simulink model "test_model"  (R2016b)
settings: Solver=VariableStepAuto  StartTime=0.0  StopTime=runtime  RelTol=1e-3
InitFcn:
  | clear mex
  | delete test_model_sfun.mexw64
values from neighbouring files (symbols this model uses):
  delta_T = 4 * [ 0,  0,  2.351e-4 ]    [modelParameters.m]
  Delta_T = cell(1,4)    [modelParameters.m]
  F_D = 1*randn(3,1)    [modelParameters.m]
  g = 9.81    [modelParameters.m]    (also in analyzeIMU_data.m = 9.8; getMomentOfInertia.m = 9.80665)
  Gamma_H = cell(1,4)    [modelParameters.m]
  have_motor_transient = 1    [modelParameters.m]
  height_controlled_o = (((Rm*If        + (((omega0_o * 2 * Rm * Kv * Kq      * Kd + 1)^2) - 1)/(4* Rm*Kv^2*Kq      * Kd))/Vb)*(Pmax - Pmin) + Pmin)    [modelParameters.m]
  i_0 = cell(1,4)    [modelParameters.m]
  If = 0.3836    [modelParameters.m]    (also in thrustDragConstantCalculations.m = [If0; If1; If2; If3]; Kd_error.m = I_0 * sign(rotor_speed_0) + I_1 * rotor_speed_0 + I_2 * roto)
  J = diag([ 0.0130 0.0140 0.0285 ])    [modelParameters.m]    (also in J_calc_bifilar.m = (16*pi^2*L./(m*g.*D.^2))\(t./n).^2)
  J_L = m_L/12*diag([y_L^2+z_L^2,x_L^2+z_L^2,x_L^2+y_L^2])    [modelParameters.m]
  J_r = cell(1,4)    [modelParameters.m]
  Jreq = 4.2012e-05    [modelParameters.m]
  Jxx = 0.0130    (= 0.013)    [modelParameters.m]
  Jyy = 0.0140    (= 0.014)    [modelParameters.m]
  Jzz = 0.0285    [modelParameters.m]
  K_d = cell(1,4)    [modelParameters.m]
  K_E = cell(1,4)    [modelParameters.m]
  K_H = cell(1,4)    [modelParameters.m]
  K_Q = cell(1,4)    [modelParameters.m]
  K_T = cell(1,4)    [modelParameters.m]
  K_V = cell(1,4)    [modelParameters.m]
  Kd = 1.4852e-07    [modelParameters.m]    (also in calcDragConstant.m = ((A'*A)^-1)*A'*b; thrustDragConstantCalculations.m = calcDragConstant(data, Pmin, Pmax, Rm, Kv, Kq, If); Kd_error.m = 1.0317e-07)
  Kh = 3.4574e-04    (= 0.00034574)    [modelParameters.m]
  Ki_mahony = 0.001    [modelParameters.m]
  Kp_mahony = 0.4    [modelParameters.m]
  Kq = 96.3422    [modelParameters.m]    (also in thrustDragConstantCalculations.m; Kd_error.m)
  Kt = 1.2007e-05    [modelParameters.m]    (also in calcThrustConstant.m = ((A'*A)^(-1))*(A'*T); thrustDragConstantCalculations.m = calcThrustConstant(data))
  Kv = 96.3422    [modelParameters.m]    (also in thrustDragConstantCalculations.m; Kd_error.m)
  m = 1.216    [modelParameters.m]
  m_L = 0    [modelParameters.m]
  omega0_o = sqrt((m*g)/(4*Kt))    [modelParameters.m]
  omega1_o = sqrt((m*g)/(4*Kt))    [modelParameters.m]
  omega2_o = sqrt((m*g)/(4*Kt))    [modelParameters.m]
  omega3_o = sqrt((m*g)/(4*Kt))    [modelParameters.m]
  omega_0 = cell(1,4)    [modelParameters.m]
  p0 = 0    [modelParameters.m]
  p_0 = cell(1,4)    [modelParameters.m]
  p_max = cell(1,4)    [modelParameters.m]
  phi0 = 0    [modelParameters.m]
  pitch_o = 0    [modelParameters.m]
  pitchrate_o = 0    [modelParameters.m]
  Pmax = 1    [modelParameters.m]    (also in thrustDragConstantCalculations.m = 200000; Kd_error.m = 200000)
  Pmin = 0    [modelParameters.m]    (also in thrustDragConstantCalculations.m = 100000; Kd_error.m = 100000)
  psi0 = 0    [modelParameters.m]
  q0 = 0    [modelParameters.m]
  Q_D = 0.05*randn(3,1)    [modelParameters.m]
  r0 = 0    [modelParameters.m]
  R_m = cell(1,4)    [modelParameters.m]
  r_oc = [ 0 ; 0 ; 0 ]    [modelParameters.m]
  r_oL = [0; 0; 0]    [modelParameters.m]
  rhx = 0.16    [modelParameters.m]
  rhy = 0.16    [modelParameters.m]
  rhz = 0.03    [modelParameters.m]
  Rm = 0.235    [modelParameters.m]    (also in thrustDragConstantCalculations.m = 0.2308; Kd_error.m = 0.2308)
  roll_o = 0    [modelParameters.m]
  rollrate_o = 0    [modelParameters.m]
  Tc = 0.04    [modelParameters.m]
  theta0 = 0    [modelParameters.m]
  Tq = 0.005    [modelParameters.m]
  u0 = 0    [modelParameters.m]
  v0 = 0    [modelParameters.m]
  Vb = 12.3    [modelParameters.m]    (also in calcDragConstant.m = [data.(6); data.(6); data.(6); data.(6)]; Kd_error.m = data.(6))
  w0 = 0    [modelParameters.m]
  x0 = 0    [modelParameters.m]
  x_controlled_o = 0    [modelParameters.m]
  x_o = 0    [modelParameters.m]
  x_vel_o = 0    [modelParameters.m]
  y0 = 0    [modelParameters.m]
  y_controlled_o = 0    [modelParameters.m]
  y_o = 0    [modelParameters.m]
  y_vel_o = 0    [modelParameters.m]
  yaw_controlled_o = 0    [modelParameters.m]
  yaw_o = 0    [modelParameters.m]
  yawrate_o = 0    [modelParameters.m]
  z0 = 0    [modelParameters.m]
  z_o = 0    [modelParameters.m]
  z_vel_o = 0    [modelParameters.m]
undefined symbols (not defined in the file or in its folder): Gamma_Omega, Gamma_T, Ki, Kp, r_h, slope, start, Ts, X0
libraries: simulink x32, Derivative x26, dsparch4 x6, vrlib x4
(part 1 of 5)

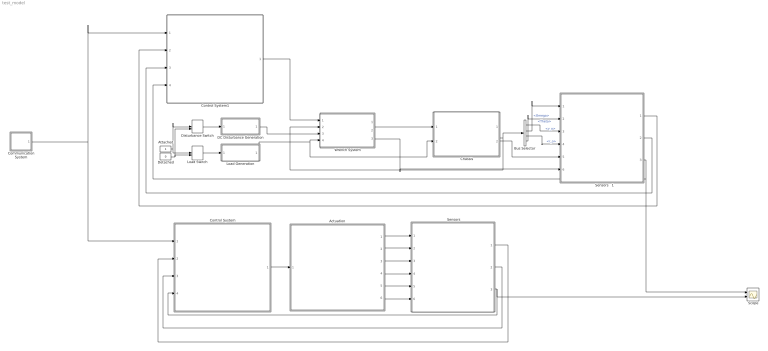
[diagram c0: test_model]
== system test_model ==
  "     Sensors   " : Subsystem
  "     Sensors   1" : Subsystem
  Actuation : Subsystem
  Attached : Constant
  Bus Selector : BusSelector  OutputSignals=v_o,Omega,r_o,Theta
  Chassis : Subsystem
  Communication System : Subsystem
  Control System : Subsystem
  Control System1 : Subsystem
  DC Disturbance Generation : Subsystem
  Detached : Constant  Value=0
  Disturbance Switch : ManualSwitch  CurrentSetting=0
  Load Generation : Subsystem
  Load Switch : ManualSwitch  CurrentSetting=0
  Scope : Scope  NumInputPorts=2
  Wrench System : Subsystem
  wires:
  Communication System/1(setpoints) -> Control System1/1(setpoints), Control System/1(setpoints)
  Wrench System/1(W) -> Chassis/1(W)
  Load Generation/1(Load) -> Chassis/2(Load), Wrench System/4(Load)
  DC Disturbance Generation/1(Disturbance) -> Wrench System/3(W_D)
  Attached/1 -> Load Switch/1, Disturbance Switch/1
  Detached/1 -> Load Switch/2, Disturbance Switch/2
  Load Switch/1 -> Load Generation/1(On/Off)
  Disturbance Switch/1 -> DC Disturbance Generation/1(On/Off)
  Chassis/1(Lambda) -> Wrench System/2(Lambda), Bus Selector/1
  Control System1/1(P) -> Wrench System/1(P)
  Control System/1(P) -> Actuation/1(P)
  Actuation/6(B_g) -> "     Sensors   "/6(B_g)
  Actuation/5(B_vo_dot) -> "     Sensors   "/5(B_vo_dot)
  Actuation/4(E_ro) -> "     Sensors   "/4(E_ro)
  Actuation/3(B_vo) -> "     Sensors   "/3(B_vo)
  Actuation/1(B_omega) -> "     Sensors   "/1(B_Omega)
  "     Sensors   "/3(current_position) -> Control System/4(current_position), Scope/2
  "     Sensors   "/2(euler_rates) -> Control System/3(euler_rates)
  "     Sensors   "/1(euler_angles_filtered) -> Control System/2(euler_angles_filtered)
  Bus Selector/1 -> "     Sensors   1"/3(B_vo)  "<v_o>"
  Bus Selector/2 -> "     Sensors   1"/1(B_Omega)  "<Omega>"
  Bus Selector/3 -> "     Sensors   1"/4(E_ro)  "<r_o>"
  Bus Selector/4 -> "     Sensors   1"/2(euler_angles)  "<Theta>"
  Chassis/2(B_vo_dot) -> "     Sensors   1"/5(B_vo_dot)
  Wrench System/3(Bg) -> "     Sensors   1"/6(B_g)
  "     Sensors   1"/3(current_position) -> Control System1/4(current_position), Scope/1
  "     Sensors   1"/2(euler_rates) -> Control System1/3(euler_rates)
  "     Sensors   1"/1(euler_angles_filtered) -> Control System1/2(euler_angles_filtered)
  Actuation/2(euler_angles) -> "     Sensors   "/2(euler_angles)

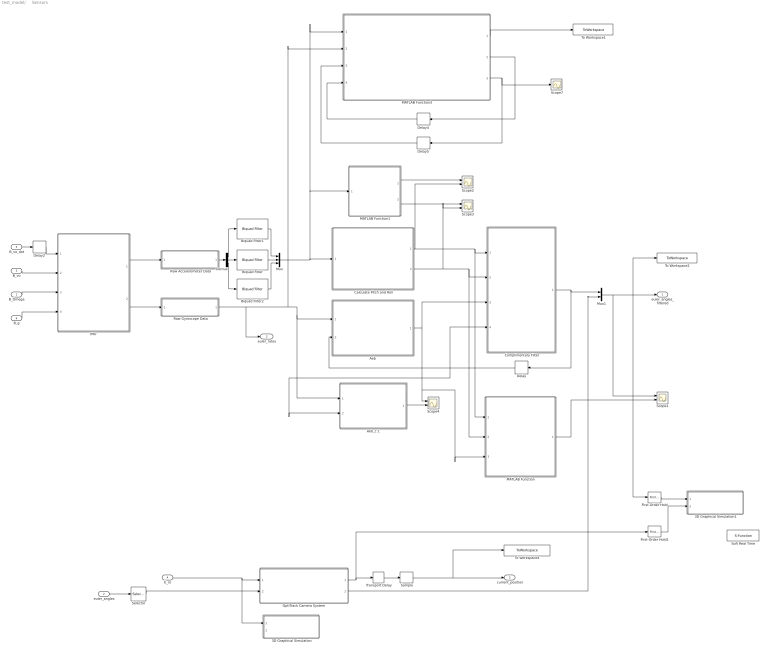
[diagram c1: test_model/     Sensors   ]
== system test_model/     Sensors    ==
  B_Omega : Inport
  euler_angles : Inport  Port=2
  B_vo : Inport  Port=3
  E_ro : Inport  Port=4
  B_vo_dot : Inport  Port=5
  B_g : Inport  Port=6
  3D Graphical Simulation : Subsystem  Commented=on
  3D Graphical Simulation1 : Subsystem  Commented=on
  "Aeb " : MATLAB Function  TreatAsAtomicUnit=on
  Aeb_c 1 : MATLAB Function  TreatAsAtomicUnit=on
  Biquad Filter : dsparch4/Biquad Filter  IIRFiltStruct=Direct form II  CoeffSource=Specify via dialog  BiQuadCoeffs=SOS_Matrix  a0Flag=Warning  IC=0  ICnum=0  ICden=0  InputProcessing=Columns as channels (frame based)  denAccumFracLength=30  denProdOutputFracLength=30  secondMemoryFracLength=15  roundingMode=Floor  overflowMode=off  ScaleValues=1  optimizeScaleValues=on  ScaleValueMode=Specify via input port (g)  scaleValueFracLength=14  FilterSource=Specify via dialog  FilterObject=BQF
  Biquad Filter1 : dsparch4/Biquad Filter  IIRFiltStruct=Direct form II  CoeffSource=Specify via dialog  BiQuadCoeffs=SOS_Matrix  a0Flag=Warning  IC=0  ICnum=0  ICden=0  InputProcessing=Columns as channels (frame based)  denAccumFracLength=30  denProdOutputFracLength=30  secondMemoryFracLength=15  roundingMode=Floor  overflowMode=off  ScaleValues=1  optimizeScaleValues=on  ScaleValueMode=Specify via input port (g)  scaleValueFracLength=14  FilterSource=Specify via dialog  FilterObject=BQF
  Biquad Filter2 : dsparch4/Biquad Filter  IIRFiltStruct=Direct form II  CoeffSource=Specify via dialog  BiQuadCoeffs=SOS_Matrix  a0Flag=Warning  IC=0  ICnum=0  ICden=0  InputProcessing=Columns as channels (frame based)  denAccumFracLength=30  denProdOutputFracLength=30  secondMemoryFracLength=15  roundingMode=Floor  overflowMode=off  ScaleValues=1  optimizeScaleValues=on  ScaleValueMode=Specify via input port (g)  scaleValueFracLength=14  FilterSource=Specify via dialog  FilterObject=BQF
  Calculate Pitch and Roll : MATLAB Function  TreatAsAtomicUnit=on
  Complimentary Filter : MATLAB Function  TreatAsAtomicUnit=on
  Delay : Delay  DelayLength=1  InitialCondition=0
  Delay2 : Delay  DelayLength=1  InitialCondition=0  SampleTime=Tq
  Delay4 : Delay  DelayLength=1  InitialCondition=0  SampleTime=Tq
  Delay5 : Delay  DelayLength=1  InitialCondition=[1, 0, 0, 0]  SampleTime=Tq
  Demux : Demux  Outputs=3
  First-Order Hold : simulink/Discrete/First-Order Hold  DisableCoverage=on  Ts=5e-3
  First-Order Hold1 : simulink/Discrete/First-Order Hold  DisableCoverage=on  Ts=5e-3
  "IMU " : Subsystem
  MATLAB Function : MATLAB Function  TreatAsAtomicUnit=on
  MATLAB Function1 : MATLAB Function  TreatAsAtomicUnit=on
  MATLAB Function3 : MATLAB Function  TreatAsAtomicUnit=on
  Mux : Mux  Inputs=3
  Mux1 : Mux  Inputs=2
  "OptiTrack Camera System " : Subsystem
  Raw Accelerometer Data : Subsystem  Variant=on
  Raw Gyroscope Data : Subsystem  Variant=on
  Sample : ZeroOrderHold  SampleTime=Tc
  Scope{1..4} (4 alike) : Scope  NumInputPorts=2
  Scope7 : Scope
  Selector : Selector  InputPortWidth=3  IndexOptions=Index vector (dialog)  Indices=[3]  OutputSizes=1
  Soft Real Time : S-Function  Commented=on  FunctionName=sfun_time  Parameters=x  SFunctionDeploymentMode=off  EnableBusSupport=off
  To Workspace1 : ToWorkspace  VariableName=mahony_reading  SaveFormat=Structure With Time  SampleTime=Tq
  To Workspace2 : ToWorkspace  VariableName=angle_IMU_reading  SaveFormat=Structure With Time  SampleTime=Tq
  To Workspace4 : ToWorkspace  VariableName=position_model  SaveFormat=Structure With Time  SampleTime=Tc
  Transport Delay : TransportDelay  DelayTime=6e-3
  euler_angles_filtered : Outport
  euler_rates : Outport  Port=2
  current_position : Outport  Port=3
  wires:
  "IMU "/1(accelerometer) -> Raw Accelerometer Data/1(raw_accel_model)
  "IMU "/2(gyroscope) -> Raw Gyroscope Data/1(raw_gyro_model)
  B_vo/1 -> "IMU "/2(B_vo)
  B_Omega/1 -> "IMU "/3(B_Omega)
  B_g/1 -> "IMU "/4(B_g)
  Calculate Pitch and Roll/2(accel_roll) -> Scope3/2, MATLAB Function/2(accel_roll), Complimentary Filter/2(accel_roll)
  Calculate Pitch and Roll/1(accel_pitch) -> MATLAB Function/1(accel_pitch), Complimentary Filter/1(accel_pitch), Scope2/2
  First-Order Hold/1 -> 3D Graphical Simulation1/1("Euler Angles ")
  E_ro/1 -> 3D Graphical Simulation/1(Displacement), "OptiTrack Camera System "/1(E_ro)
  First-Order Hold1/1 -> 3D Graphical Simulation1/2(Displacement)
  B_vo_dot/1 -> Delay2/1
  Delay2/1 -> "IMU "/1(B_vo_dot)
  "OptiTrack Camera System "/1(E_ro_camera) -> Transport Delay/1, First-Order Hold1/1
  Transport Delay/1 -> Sample/1
  Sample/1 -> To Workspace4/1, current_position/1
  Raw Gyroscope Data/1(raw_gyro) -> Aeb_c 1/1(gyro_reading), "Aeb "/1(gyro_reading), MATLAB Function3/2(gyroReadings), euler_rates/1
  Delay/1 -> Complimentary Filter/4(prev_euler_angles), Aeb_c 1/2(euler_angles_filtered), "Aeb "/2(euler_angles_filtered)
  Aeb_c 1/1(euler_rates_IMU) -> Scope4/2
  MATLAB Function1/1(accel_pitch) -> Scope2/1
  MATLAB Function1/2(accel_roll) -> Scope3/1
  "OptiTrack Camera System "/2(yaw_camera) -> Mux1/2
  MATLAB Function3/1(eulerAngles) -> To Workspace1/1
  MATLAB Function3/2(integralFeedback) -> Delay4/1
  Delay4/1 -> MATLAB Function3/4(integralFeedback_prev)
  MATLAB Function3/3(quaternions) -> Scope7/1, Delay5/1
  Delay5/1 -> MATLAB Function3/3(quaternions_prev)
  "Aeb "/1(euler_rates_IMU) -> MATLAB Function/3(euler_rates_gyro), Scope4/1, Complimentary Filter/3(euler_rates_gyro)
  Raw Accelerometer Data/1(raw_accel) -> Demux/1
  Demux/2 -> Biquad Filter/1
  Demux/1 -> Biquad Filter1/1
  Demux/3 -> Biquad Filter2/1
  Biquad Filter/1 -> Mux/2
  Biquad Filter1/1 -> Mux/1
  Biquad Filter2/1 -> Mux/3
  Mux/1 -> Calculate Pitch and Roll/1(accel_reading), MATLAB Function1/1(accel_reading), MATLAB Function3/1(accelReadings)
  Complimentary Filter/1(euler_angles_IMU) -> Mux1/1, Delay/1
  euler_angles/1 -> Selector/1
  Selector/1 -> "OptiTrack Camera System "/2(yaw)
  MATLAB Function/1(euler_angles_IMU) -> Scope1/2
  Mux1/1 -> Scope1/1, To Workspace2/1, First-Order Hold/1, euler_angles_filtered/1

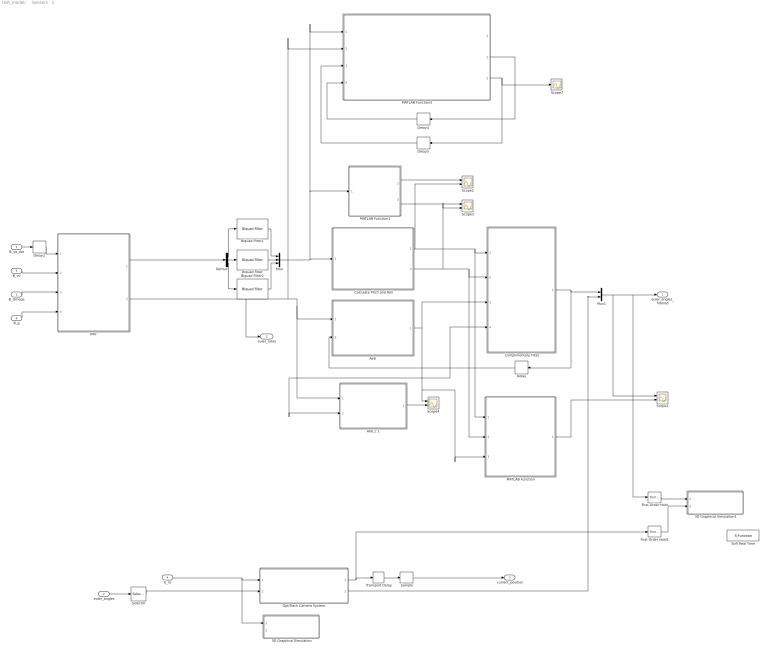
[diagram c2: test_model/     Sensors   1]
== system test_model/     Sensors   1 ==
  B_Omega : Inport
  euler_angles : Inport  Port=2
  B_vo : Inport  Port=3
  E_ro : Inport  Port=4
  B_vo_dot : Inport  Port=5
  B_g : Inport  Port=6
  3D Graphical Simulation : Subsystem  Commented=on
  3D Graphical Simulation1 : Subsystem  Commented=on
  "Aeb " : MATLAB Function  TreatAsAtomicUnit=on
  Aeb_c 1 : MATLAB Function  TreatAsAtomicUnit=on
  Biquad Filter : dsparch4/Biquad Filter  IIRFiltStruct=Direct form II  CoeffSource=Specify via dialog  BiQuadCoeffs=SOS_Matrix  a0Flag=Warning  IC=0  ICnum=0  ICden=0  InputProcessing=Columns as channels (frame based)  denAccumFracLength=30  denProdOutputFracLength=30  secondMemoryFracLength=15  roundingMode=Floor  overflowMode=off  ScaleValues=1  optimizeScaleValues=on  ScaleValueMode=Specify via input port (g)  scaleValueFracLength=14  FilterSource=Specify via dialog  FilterObject=BQF
  Biquad Filter1 : dsparch4/Biquad Filter  IIRFiltStruct=Direct form II  CoeffSource=Specify via dialog  BiQuadCoeffs=SOS_Matrix  a0Flag=Warning  IC=0  ICnum=0  ICden=0  InputProcessing=Columns as channels (frame based)  denAccumFracLength=30  denProdOutputFracLength=30  secondMemoryFracLength=15  roundingMode=Floor  overflowMode=off  ScaleValues=1  optimizeScaleValues=on  ScaleValueMode=Specify via input port (g)  scaleValueFracLength=14  FilterSource=Specify via dialog  FilterObject=BQF
  Biquad Filter2 : dsparch4/Biquad Filter  IIRFiltStruct=Direct form II  CoeffSource=Specify via dialog  BiQuadCoeffs=SOS_Matrix  a0Flag=Warning  IC=0  ICnum=0  ICden=0  InputProcessing=Columns as channels (frame based)  denAccumFracLength=30  denProdOutputFracLength=30  secondMemoryFracLength=15  roundingMode=Floor  overflowMode=off  ScaleValues=1  optimizeScaleValues=on  ScaleValueMode=Specify via input port (g)  scaleValueFracLength=14  FilterSource=Specify via dialog  FilterObject=BQF
  Calculate Pitch and Roll : MATLAB Function  TreatAsAtomicUnit=on
  Complimentary Filter : MATLAB Function  TreatAsAtomicUnit=on
  Delay : Delay  DelayLength=1  InitialCondition=0
  Delay2 : Delay  DelayLength=1  InitialCondition=0  SampleTime=Tq
  Delay4 : Delay  DelayLength=1  InitialCondition=0  SampleTime=Tq
  Delay5 : Delay  DelayLength=1  InitialCondition=[1, 0, 0, 0]  SampleTime=Tq
  Demux : Demux  Outputs=3
  First-Order Hold : simulink/Discrete/First-Order Hold  DisableCoverage=on  Ts=5e-3
  First-Order Hold1 : simulink/Discrete/First-Order Hold  DisableCoverage=on  Ts=5e-3
  "IMU " : Subsystem
  MATLAB Function : MATLAB Function  TreatAsAtomicUnit=on
  MATLAB Function1 : MATLAB Function  TreatAsAtomicUnit=on
  MATLAB Function3 : MATLAB Function  TreatAsAtomicUnit=on
  Mux : Mux  Inputs=3
  Mux1 : Mux  Inputs=2
  "OptiTrack Camera System " : Subsystem
  Sample : ZeroOrderHold  SampleTime=Tc
  Scope{1..4} (4 alike) : Scope  NumInputPorts=2
  Scope7 : Scope
  Selector : Selector  InputPortWidth=3  IndexOptions=Index vector (dialog)  Indices=[3]  OutputSizes=1
  Soft Real Time : S-Function  Commented=on  FunctionName=sfun_time  Parameters=x  SFunctionDeploymentMode=off  EnableBusSupport=off
  Transport Delay : TransportDelay  DelayTime=6e-3
  euler_angles_filtered : Outport
  euler_rates : Outport  Port=2
  current_position : Outport  Port=3
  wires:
  B_vo/1 -> "IMU "/2(B_vo)
  B_Omega/1 -> "IMU "/3(B_Omega)
  B_g/1 -> "IMU "/4(B_g)
  Calculate Pitch and Roll/2(accel_roll) -> Scope3/2, MATLAB Function/2(accel_roll), Complimentary Filter/2(accel_roll)
  Calculate Pitch and Roll/1(accel_pitch) -> MATLAB Function/1(accel_pitch), Complimentary Filter/1(accel_pitch), Scope2/2
  First-Order Hold/1 -> 3D Graphical Simulation1/1("Euler Angles ")
  E_ro/1 -> 3D Graphical Simulation/1(Displacement), "OptiTrack Camera System "/1(E_ro)
  First-Order Hold1/1 -> 3D Graphical Simulation1/2(Displacement)
  B_vo_dot/1 -> Delay2/1
  Delay2/1 -> "IMU "/1(B_vo_dot)
  "OptiTrack Camera System "/1(E_ro_camera) -> Transport Delay/1, First-Order Hold1/1
  Transport Delay/1 -> Sample/1
  Sample/1 -> current_position/1
  "IMU "/2(gyroscope) -> Aeb_c 1/1(gyro_reading), "Aeb "/1(gyro_reading), MATLAB Function3/2(gyroReadings), euler_rates/1
  Delay/1 -> Complimentary Filter/4(prev_euler_angles), Aeb_c 1/2(euler_angles_filtered), "Aeb "/2(euler_angles_filtered)
  Aeb_c 1/1(euler_rates_IMU) -> Scope4/2
  MATLAB Function1/1(accel_pitch) -> Scope2/1
  MATLAB Function1/2(accel_roll) -> Scope3/1
  "OptiTrack Camera System "/2(yaw_camera) -> Mux1/2
  MATLAB Function3/2(integralFeedback) -> Delay4/1
  Delay4/1 -> MATLAB Function3/4(integralFeedback_prev)
  MATLAB Function3/3(quaternions) -> Scope7/1, Delay5/1
  Delay5/1 -> MATLAB Function3/3(quaternions_prev)
  "Aeb "/1(euler_rates_IMU) -> MATLAB Function/3(euler_rates_gyro), Scope4/1, Complimentary Filter/3(euler_rates_gyro)
  "IMU "/1(accelerometer) -> Demux/1
  Demux/2 -> Biquad Filter/1
  Demux/1 -> Biquad Filter1/1
  Demux/3 -> Biquad Filter2/1
  Biquad Filter/1 -> Mux/2
  Biquad Filter1/1 -> Mux/1
  Biquad Filter2/1 -> Mux/3
  Mux/1 -> Calculate Pitch and Roll/1(accel_reading), MATLAB Function1/1(accel_reading), MATLAB Function3/1(accelReadings)
  Complimentary Filter/1(euler_angles_IMU) -> Mux1/1, Delay/1
  euler_angles/1 -> Selector/1
  Selector/1 -> "OptiTrack Camera System "/2(yaw)
  MATLAB Function/1(euler_angles_IMU) -> Scope1/2
  Mux1/1 -> Scope1/1, First-Order Hold/1, euler_angles_filtered/1

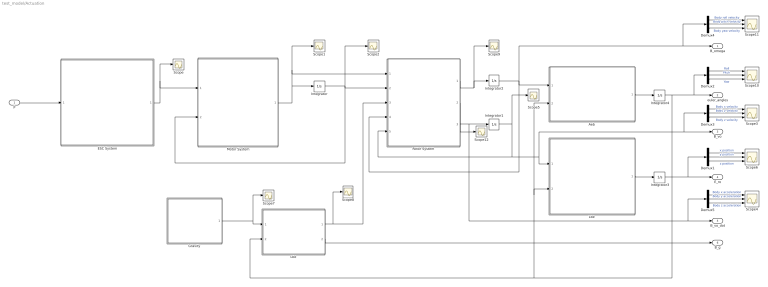
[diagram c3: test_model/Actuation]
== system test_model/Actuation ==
  P : Inport
  "Aeb " : MATLAB Function  TreatAsAtomicUnit=on
  Demux{1..5} (5 alike) : Demux  Outputs=3
  ESC System : MATLAB Function  TreatAsAtomicUnit=on
  "Gravity " : MATLAB Function  TreatAsAtomicUnit=on
  Integrator : Integrator  InitialCondition=[omega0_o, omega1_o, omega2_o, omega3_o]
  Integrator1 : Integrator  InitialCondition=[x_vel_o; y_vel_o; z_vel_o]
  Integrator2 : Integrator  InitialCondition=[rollrate_o; pitchrate_o; yawrate_o]
  Integrator3 : Integrator  InitialCondition=[x_o; y_o; z_o]
  Integrator4 : Integrator  InitialCondition=[roll_o; pitch_o; yaw_o]  ContinuousStateAttributes=['phi' 'theta' 'psi']
  "Lbe " : MATLAB Function  TreatAsAtomicUnit=on
  "Lbe " : MATLAB Function  TreatAsAtomicUnit=on
  Motor System : MATLAB Function  TreatAsAtomicUnit=on
  "Rotor System " : MATLAB Function  TreatAsAtomicUnit=on
  Scope{,1..2,5,7..9,12} (8 alike) : Scope
  Scope{3..4,6,10..11} (5 alike) : Scope  NumInputPorts=3
  B_omega : Outport
  euler_angles : Outport  Port=2
  B_vo : Outport  Port=3
  E_ro : Outport  Port=4
  B_vo_dot : Outport  Port=5
  B_g : Outport  Port=6
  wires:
  ESC System/1(Vb_eff) -> Scope/1, Motor System/1(Vb_eff)
  "Rotor System "/1(B_omega_dot) -> Scope9/1, Integrator2/1
  Integrator2/1 -> "Rotor System "/4(B_omega), B_omega/1, Demux4/1, "Aeb "/1(B_omega)
  "Aeb "/1(euler_rates) -> Integrator4/1
  "Lbe "/1(E_ro) -> Integrator3/1
  Integrator3/1 -> Demux1/1, E_ro/1
  "Lbe "/1(B_Fg) -> Scope8/1, "Rotor System "/3(B_Fg)
  "Lbe "/2(B_g) -> B_g/1
  Demux1/2 -> Scope6/2  "y position"
  Demux1/1 -> Scope6/1  "x position"
  Demux1/3 -> Scope6/3  "z position"
  Demux2/2 -> Scope10/2  "Pitch"
  Demux2/1 -> Scope10/1  "Roll"
  Demux2/3 -> Scope10/3  "Yaw"
  Demux4/2 -> Scope11/2  "Body pitch velocity"
  Demux4/1 -> Scope11/1  "Body roll velocity"
  Demux4/3 -> Scope11/3  "Body yaw velocity"
  Demux3/2 -> Scope3/2  "Body y velocity"
  Demux3/1 -> Scope3/1  "Body x velocity"
  Demux3/3 -> Scope3/3  "Body z velocity"
  Demux5/2 -> Scope4/2  "Body y acceleration"
  Demux5/1 -> Scope4/1  "Body x acceleration"
  Demux5/3 -> Scope4/3  "Body z acceleration"
  Integrator1/1 -> Scope5/1, "Rotor System "/5(B_vo), "Lbe "/1(B_vo), Demux3/1, B_vo/1
  "Rotor System "/2(B_vo_dot) -> Demux5/1, B_vo_dot/1, Integrator1/1
  Integrator4/1 -> euler_angles/1, Demux2/1, "Lbe "/2(euler_angles), "Aeb "/2(euler_angles), "Lbe "/2(euler_angles)
  P/1 -> ESC System/1(P)
  "Gravity "/1(E_Fg) -> Scope7/1, "Lbe "/1(E_Fg)
  Integrator/1 -> Motor System/2(w), "Rotor System "/2(w), Scope2/1
  Motor System/1(w_dot) -> Integrator/1, Scope1/1, "Rotor System "/1(w_dot)
  "Rotor System "/3(B_F) -> Scope12/1

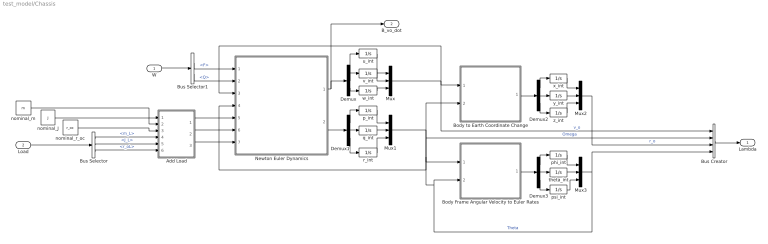
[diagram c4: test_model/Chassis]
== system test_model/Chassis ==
  W : Inport
  Load : Inport  Port=2
  Add Load : Subsystem
  Body Frame Angular Velocity to Euler Rates : MATLAB Function  TreatAsAtomicUnit=on
  Body to Earth Coordinate Change : MATLAB Function  TreatAsAtomicUnit=on
  Bus Creator : BusCreator  Inputs=4
  Bus Selector : BusSelector  OutputSignals=m_L,J_L,r_oL
  Bus Selector1 : BusSelector  OutputSignals=F,Q
  Demux{,1..3} (4 alike) : Demux  Outputs=3
  Mux{,1..3} (4 alike) : Mux  Inputs=3
  Newton Euler Dynamics : Subsystem
  nominal_J : Constant  Value=J
  nominal_m : Constant  Value=m
  nominal_r_oc : Constant  Value=r_oc
  p_int : Integrator  InitialCondition=p0  ContinuousStateAttributes='p'
  phi_int : Integrator  InitialCondition=phi0  ContinuousStateAttributes='phi'
  psi_int : Integrator  InitialCondition=psi0  ContinuousStateAttributes='psi'
  q_int : Integrator  InitialCondition=q0  ContinuousStateAttributes='q'
  r_int : Integrator  InitialCondition=r0  ContinuousStateAttributes='r'
  theta_int : Integrator  InitialCondition=theta0  ContinuousStateAttributes='theta'
  u_int : Integrator  InitialCondition=u0  ContinuousStateAttributes='u'
  v_int : Integrator  InitialCondition=v0  ContinuousStateAttributes='v'
  w_int : Integrator  InitialCondition=w0  ContinuousStateAttributes='w'
  x_int : Integrator  InitialCondition=x0  ContinuousStateAttributes='x'
  y_int : Integrator  InitialCondition=y0  ContinuousStateAttributes='y'
  z_int : Integrator  InitialCondition=z0  ContinuousStateAttributes='z'
  Lambda : Outport
  B_vo_dot : Outport  Port=2
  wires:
  nominal_J/1 -> Add Load/2(J_0)
  Bus Selector/3 -> Add Load/6(r_ol)  "<r_oL>"
  Bus Selector/2 -> Add Load/5(J_l)  "<J_L>"
  Bus Selector/1 -> Add Load/4(m_l)  "<m_L>"
  Add Load/3(r_oc) -> Newton Euler Dynamics/7(r_oc)
  Add Load/2(J) -> Newton Euler Dynamics/6(J)
  Add Load/1(m) -> Newton Euler Dynamics/5(m)
  W/1 -> Bus Selector1/1
  Bus Selector1/2 -> Newton Euler Dynamics/2(Q)  "<Q>"
  Bus Selector1/1 -> Newton Euler Dynamics/1(F)  "<F>"
  Body Frame Angular Velocity to Euler Rates/1(dot_Theta) -> Demux3/1
  Demux3/3 -> psi_int/1
  Demux3/2 -> theta_int/1
  Demux3/1 -> phi_int/1
  psi_int/1 -> Mux3/3
  theta_int/1 -> Mux3/2
  phi_int/1 -> Mux3/1
  Body to Earth Coordinate Change/1(x_E) -> Demux2/1
  Demux2/3 -> z_int/1
  Demux2/2 -> y_int/1
  Demux2/1 -> x_int/1
  z_int/1 -> Mux2/3
  y_int/1 -> Mux2/2
  x_int/1 -> Mux2/1
  Newton Euler Dynamics/2(dOmega) -> Demux1/1
  Demux1/3 -> r_int/1
  Demux1/2 -> q_int/1
  Demux1/1 -> p_int/1
  r_int/1 -> Mux1/3
  q_int/1 -> Mux1/2
  p_int/1 -> Mux1/1
  Newton Euler Dynamics/1(dv) -> B_vo_dot/1, Demux/1
  Demux/3 -> w_int/1
  Demux/2 -> v_int/1
  Demux/1 -> u_int/1
  w_int/1 -> Mux/3
  v_int/1 -> Mux/2
  u_int/1 -> Mux/1
  Bus Creator/1 -> Lambda/1
  Mux3/1 -> Body to Earth Coordinate Change/2(Theta), Body Frame Angular Velocity to Euler Rates/2(Theta), Bus Creator/4  "Theta"
  Mux2/1 -> Bus Creator/3  "r_o"
  Mux1/1 -> Body Frame Angular Velocity to Euler Rates/1(Omega_B), Newton Euler Dynamics/4(Omega), Bus Creator/2  "Omega"
  Mux/1 -> Bus Creator/1, Body to Earth Coordinate Change/1(x_B), Newton Euler Dynamics/3(v)  "v_o"
  nominal_m/1 -> Add Load/1(m_0)
  nominal_r_oc/1 -> Add Load/3(r_oc_0)
  Load/1 -> Bus Selector/1

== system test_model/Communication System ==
  From Workspace : FromWorkspace  VariableName=x_setpoint_model  SampleTime=Tq  Interpolate=off  OutputAfterFinalValue=Holding final value
  From Workspace1 : FromWorkspace  VariableName=z_setpoint_model  SampleTime=Tq  Interpolate=off  OutputAfterFinalValue=Holding final value
  From Workspace2 : FromWorkspace  VariableName=y_setpoint_model  SampleTime=Tq  Interpolate=off  OutputAfterFinalValue=Holding final value
  Mux : Mux
  Step : Step  Before=[0; 0; 0; 0]  After=[0; 0; 1; 0]  SampleTime=Tq
  Step1 : Step  After=0  SampleTime=0
  setpoints : Outport
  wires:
  From Workspace/1 -> Mux/1
  Mux/1 -> setpoints/1
  From Workspace2/1 -> Mux/2
  From Workspace1/1 -> Mux/3
  Step1/1 -> Mux/4

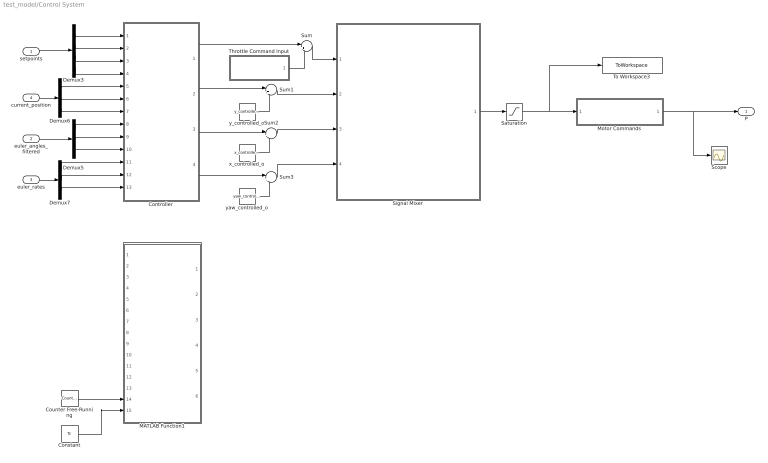
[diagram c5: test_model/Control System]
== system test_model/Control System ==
  setpoints : Inport
  euler_angles_filtered : Inport  Port=2
  euler_rates : Inport  Port=3
  current_position : Inport  Port=4
  Constant : Constant  Value=Tc  SampleTime=Tc
  Controller : Subsystem
  Counter Free-Running : simulink/Sources/Counter Free-Running  NumBits=32  tsamp=Tc
  Demux3 : Demux
  Demux5 : Demux  Outputs=3
  Demux6 : Demux  Outputs=3
  Demux7 : Demux  Outputs=3
  MATLAB Function1 : MATLAB Function  Commented=on  TreatAsAtomicUnit=on  SystemSampleTime=Tq
  Motor Commands : Subsystem  Commented=through  Variant=on
  Saturation : Saturate  UpperLimit=Pmax*ones(4,1)  LowerLimit=Pmin*ones(4,1)
  Scope : Scope
  Signal Mixer : MATLAB Function  TreatAsAtomicUnit=on
  Sum{,1..3} (4 alike) : Sum  Inputs=|++
  Throttle Command Input : Subsystem  Variant=on
  To Workspace3 : ToWorkspace  VariableName=motorCommands  SaveFormat=Structure With Time  SampleTime=Tq
  x_controlled_o : Constant  Value=x_controlled_o
  y_controlled_o : Constant  Value=y_controlled_o
  yaw_controlled_o : Constant  Value=yaw_controlled_o
  P : Outport
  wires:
  y_controlled_o/1 -> Sum1/2
  x_controlled_o/1 -> Sum2/2
  yaw_controlled_o/1 -> Sum3/2
  Signal Mixer/1(P) -> Saturation/1
  Counter Free-Running/1 -> MATLAB Function1/14(vrpn_id)
  Constant/1 -> MATLAB Function1/15(Tc)
  Sum1/1 -> Signal Mixer/2(y_controlled)
  Sum2/1 -> Signal Mixer/3(x_controlled)
  Sum3/1 -> Signal Mixer/4(yaw_controlled)
  Motor Commands/1(z_command) -> P/1, Scope/1
  Saturation/1 -> To Workspace3/1, Motor Commands/1(z_command_model)
  setpoints/1 -> Demux3/1
  current_position/1 -> Demux6/1
  euler_angles_filtered/1 -> Demux5/1
  euler_rates/1 -> Demux7/1
  Demux3/1 -> Controller/1(x_setpoint)
  Demux3/2 -> Controller/2(y_setpoint)
  Demux3/3 -> Controller/3(z_setpoint)
  Demux3/4 -> Controller/4(yaw_setpoint)
  Demux6/1 -> Controller/5(x_position)
  Demux6/2 -> Controller/6(y_position)
  Demux6/3 -> Controller/7(z_position)
  Demux5/1 -> Controller/8(roll)
  Demux5/2 -> Controller/9(pitch)
  Demux5/3 -> Controller/10(yaw)
  Demux7/1 -> Controller/11(roll_rate)
  Demux7/2 -> Controller/12(pitch_rate)
  Demux7/3 -> Controller/13(yaw_rate)
  Controller/1(height_controlled) -> Sum/1
  Controller/2(y_controlled) -> Sum1/1
  Controller/3(x_controlled) -> Sum2/1
  Controller/4(yaw_controlled) -> Sum3/1
  Throttle Command Input/1(z_command) -> Sum/2
  Sum/1 -> Signal Mixer/1(height_controlled)

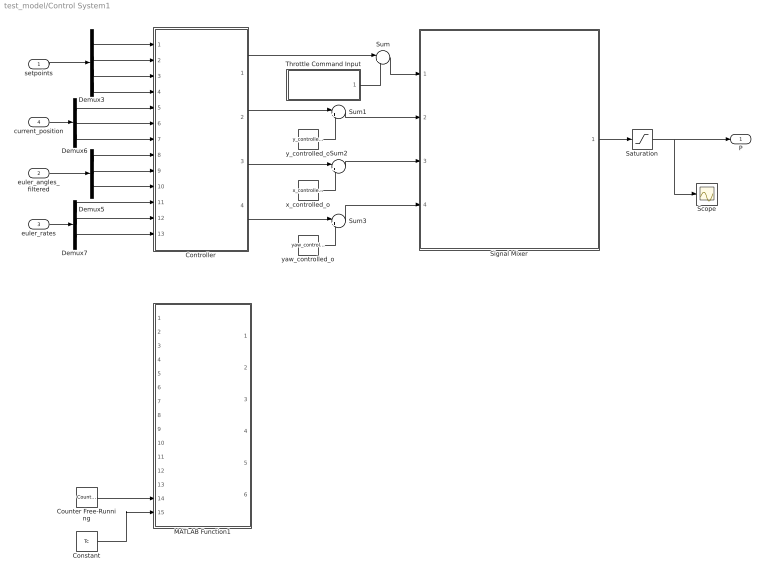
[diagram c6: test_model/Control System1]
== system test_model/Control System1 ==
  setpoints : Inport
  euler_angles_filtered : Inport  Port=2
  euler_rates : Inport  Port=3
  current_position : Inport  Port=4
  Constant : Constant  Value=Tc  SampleTime=Tc
  Controller : Subsystem
  Counter Free-Running : simulink/Sources/Counter Free-Running  NumBits=32  tsamp=Tc
  Demux3 : Demux
  Demux5 : Demux  Outputs=3
  Demux6 : Demux  Outputs=3
  Demux7 : Demux  Outputs=3
  MATLAB Function1 : MATLAB Function  Commented=on  TreatAsAtomicUnit=on  SystemSampleTime=Tq
  Saturation : Saturate  UpperLimit=Pmax*ones(4,1)  LowerLimit=Pmin*ones(4,1)
  Scope : Scope
  Signal Mixer : MATLAB Function  TreatAsAtomicUnit=on
  Sum{,1..3} (4 alike) : Sum  Inputs=|++
  Throttle Command Input : Subsystem  Variant=on
  x_controlled_o : Constant  Value=x_controlled_o
  y_controlled_o : Constant  Value=y_controlled_o
  yaw_controlled_o : Constant  Value=yaw_controlled_o
  P : Outport
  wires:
  y_controlled_o/1 -> Sum1/2
  x_controlled_o/1 -> Sum2/2
  yaw_controlled_o/1 -> Sum3/2
  Signal Mixer/1(P) -> Saturation/1
  Counter Free-Running/1 -> MATLAB Function1/14(vrpn_id)
  Constant/1 -> MATLAB Function1/15(Tc)
  Sum1/1 -> Signal Mixer/2(y_controlled)
  Sum2/1 -> Signal Mixer/3(x_controlled)
  Sum3/1 -> Signal Mixer/4(yaw_controlled)
  Saturation/1 -> P/1, Scope/1
  setpoints/1 -> Demux3/1
  current_position/1 -> Demux6/1
  euler_angles_filtered/1 -> Demux5/1
  euler_rates/1 -> Demux7/1
  Demux3/1 -> Controller/1(x_setpoint)
  Demux3/2 -> Controller/2(y_setpoint)
  Demux3/3 -> Controller/3(z_setpoint)
  Demux3/4 -> Controller/4(yaw_setpoint)
  Demux6/1 -> Controller/5(x_position)
  Demux6/2 -> Controller/6(y_position)
  Demux6/3 -> Controller/7(z_position)
  Demux5/1 -> Controller/8(roll)
  Demux5/2 -> Controller/9(pitch)
  Demux5/3 -> Controller/10(yaw)
  Demux7/1 -> Controller/11(roll_rate)
  Demux7/2 -> Controller/12(pitch_rate)
  Demux7/3 -> Controller/13(yaw_rate)
  Controller/1(height_controlled) -> Sum/1
  Controller/2(y_controlled) -> Sum1/1
  Controller/3(x_controlled) -> Sum2/1
  Controller/4(yaw_controlled) -> Sum3/1
  Throttle Command Input/1(z_command) -> Sum/2
  Sum/1 -> Signal Mixer/1(height_controlled)

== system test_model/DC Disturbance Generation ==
  On/Off : Inport
  Bus Creator2 : BusCreator  Inputs=2
  Compare To Zero : Subsystem
  F_D : Constant  Value=F_D
  Product : Product
  Product1 : Product
  Q_D : Constant  Value=Q_D
  Disturbance : Outport
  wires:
  Compare To Zero/1(y) -> Product/2, Product1/2
  On/Off/1 -> Compare To Zero/1(u)
  Q_D/1 -> Product1/1  "Q_D"
  F_D/1 -> Product/1  "F_D"
  Bus Creator2/1 -> Disturbance/1
  Product1/1 -> Bus Creator2/2  "Q_D"
  Product/1 -> Bus Creator2/1  "F_D"

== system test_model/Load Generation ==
  On/Off : Inport
  Bus Creator1 : BusCreator  Inputs=3
  Compare To Zero : Subsystem
  J_L : Constant  Value=J_L
  Product : Product
  Product1 : Product
  Product2 : Product
  m_L : Constant  Value=m_L
  r_oL : Constant  Value=r_oL
  Load : Outport
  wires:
  Compare To Zero/1(y) -> Product/2, Product1/2, Product2/2
  On/Off/1 -> Compare To Zero/1(u)
  J_L/1 -> Product1/1  "J_L"
  r_oL/1 -> Product2/1  "r_oL"
  m_L/1 -> Product/1  "m_L"
  Bus Creator1/1 -> Load/1
  Product2/1 -> Bus Creator1/3  "r_oL"
  Product1/1 -> Bus Creator1/2  "J_L"
  Product/1 -> Bus Creator1/1  "m_L"

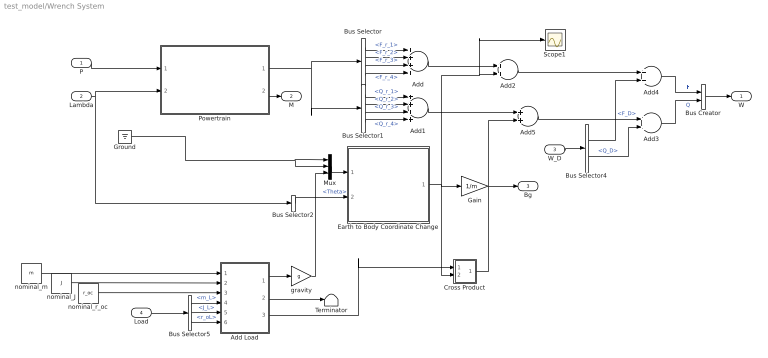
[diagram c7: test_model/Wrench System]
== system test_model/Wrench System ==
  P : Inport
  Lambda : Inport  Port=2
  W_D : Inport  Port=3
  Load : Inport  Port=4
  Add : Sum  Inputs=++++
  Add Load : Subsystem
  Add1 : Sum  Inputs=++++
  Add{2..5} (4 alike) : Sum
  Bus Creator : BusCreator  Inputs=2
  Bus Selector : BusSelector  OutputSignals=F_r_1,F_r_2,F_r_3,F_r_4
  Bus Selector1 : BusSelector  OutputSignals=Q_r_1,Q_r_2,Q_r_3,Q_r_4
  Bus Selector2 : BusSelector  OutputSignals=Theta
  Bus Selector4 : BusSelector  OutputSignals=F_D,Q_D
  Bus Selector5 : BusSelector  OutputSignals=m_L,J_L,r_oL
  Cross Product : Subsystem
  Earth to Body Coordinate Change : MATLAB Function  TreatAsAtomicUnit=on
  Gain : Gain  Gain=1/m
  Ground : Ground
  Mux : Mux  Inputs=3
  Powertrain : Subsystem
  Scope1 : Scope
  Terminator : Terminator
  gravity : Gain  Gain=g
  nominal_J : Constant  Value=J
  nominal_m : Constant  Value=m
  nominal_r_oc : Constant  Value=r_oc
  W : Outport
  M : Outport  Port=2
  Bg : Outport  Port=3
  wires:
  Add Load/2(J) -> Terminator/1
  Cross Product/1(y) -> Add5/2
  Add1/1 -> Add5/1
  Add5/1 -> Add3/1
  gravity/1 -> Mux/3
  Add Load/3(r_oc) -> Cross Product/1(a)
  Add Load/1(m) -> gravity/1
  Load/1 -> Bus Selector5/1
  Bus Selector5/3 -> Add Load/6(r_ol)  "<r_oL>"
  Bus Selector5/2 -> Add Load/5(J_l)  "<J_L>"
  Bus Selector5/1 -> Add Load/4(m_l)  "<m_L>"
  nominal_r_oc/1 -> Add Load/3(r_oc_0)
  nominal_J/1 -> Add Load/2(J_0)
  nominal_m/1 -> Add Load/1(m_0)
  Mux/1 -> Earth to Body Coordinate Change/1(x_E)
  Ground/1 -> Mux/2, Mux/1
  Powertrain/2(M) -> M/1
  W_D/1 -> Bus Selector4/1
  Bus Creator/1 -> W/1
  Add3/1 -> Bus Creator/2  "Q"
  Add4/1 -> Bus Creator/1  "F"
  Bus Selector4/2 -> Add3/2  "<Q_D>"
  Bus Selector4/1 -> Add4/2  "<F_D>"
  Add2/1 -> Add4/1
  Earth to Body Coordinate Change/1(x_B) -> Gain/1, Cross Product/2(b), Scope1/1, Add2/2
  Add/1 -> Add2/1
  Bus Selector2/1 -> Earth to Body Coordinate Change/2(Theta)  "<Theta>"
  Powertrain/1(W_r) -> Bus Selector1/1, Bus Selector/1
  Bus Selector/1 -> Add/1  "<F_r_1>"
  Bus Selector/2 -> Add/2  "<F_r_2>"
  Bus Selector/3 -> Add/3  "<F_r_3>"
  Bus Selector/4 -> Add/4  "<F_r_4>"
  Bus Selector1/1 -> Add1/1  "<Q_r_1>"
  Bus Selector1/2 -> Add1/2  "<Q_r_2>"
  Bus Selector1/3 -> Add1/3  "<Q_r_3>"
  Bus Selector1/4 -> Add1/4  "<Q_r_4>"
  P/1 -> Powertrain/1(P)
  Lambda/1 -> Bus Selector2/1, Powertrain/2(Lambda)
  Gain/1 -> Bg/1

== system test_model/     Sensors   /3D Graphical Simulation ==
  Displacement : Inport
  Euler Angles : Inport  Port=2
  Bus Creator : BusCreator  Inputs=3
  Bus Creator1 : BusCreator  Inputs=3
  Bus Creator2 : BusCreator  Inputs=3
  Bus Selector : BusSelector  OutputSignals=phi,theta,psi
  Demux : Demux  Outputs=3
  Demux1 : Demux  Outputs=3
  Gain : Gain  Gain=-1
  Gain1 : Gain  Gain=eye(3)*1  Multiplication=Matrix(K*u)
  Gain2 : Gain  Gain=-1
  MATLAB Function : MATLAB Function  TreatAsAtomicUnit=on
  Rate Transition : RateTransition  OutPortSampleTime=0.06
  Rate Transition1 : RateTransition  OutPortSampleTime=0.06
  VR Sink : vrlib/VR Sink  InstantiateOnLoad=on  SampleTime=-1  ViewEnable=on  RemoteChange=off  RemoteView=off  FieldsWritten=Helicopter.rotation.4.1.1.double#Helicopter.translation.3.1.1.double  WorldFileName=quadrotor_world_ucart.wrl  AutoView=on  VideoDimensions=[]  AllowVariableSize=off
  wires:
  Displacement/1 -> Demux/1
  Bus Creator2/1 -> Bus Selector/1
  Demux/1 -> Bus Creator1/3
  Gain/1 -> Bus Creator1/2
  Gain2/1 -> Bus Creator1/1
  Rate Transition1/1 -> VR Sink/2
  Rate Transition/1 -> VR Sink/1
  Demux/3 -> Gain/1
  Demux/2 -> Gain2/1
  Bus Creator1/1 -> Gain1/1
  Bus Selector/1 -> Bus Creator/3  "<phi>"
  Bus Selector/3 -> Bus Creator/2  "<psi>"
  Bus Selector/2 -> Bus Creator/1  "<theta>"
  Gain1/1 -> Rate Transition1/1
  Demux1/3 -> Bus Creator2/3  "psi"
  Demux1/2 -> Bus Creator2/2  "theta"
  Demux1/1 -> Bus Creator2/1  "phi"
  Euler Angles/1 -> Demux1/1
  Bus Creator/1 -> MATLAB Function/1(u)
  MATLAB Function/1(y) -> Rate Transition/1

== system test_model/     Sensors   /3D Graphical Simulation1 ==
  "Euler Angles " : Inport
  Displacement : Inport  Port=2
  Bus Creator : BusCreator  Inputs=3
  Bus Creator1 : BusCreator  Inputs=3
  Bus Creator2 : BusCreator  Inputs=3
  Bus Selector : BusSelector  OutputSignals=phi,theta,psi
  Demux : Demux  Outputs=3
  Demux1 : Demux  Outputs=3
  Gain : Gain  Gain=-1
  Gain1 : Gain  Gain=eye(3)*1  Multiplication=Matrix(K*u)
  Gain2 : Gain  Gain=-1
  MATLAB Function : MATLAB Function  TreatAsAtomicUnit=on
  Rate Transition : RateTransition  OutPortSampleTime=0.06
  Rate Transition1 : RateTransition  OutPortSampleTime=0.06
  VR Sink : vrlib/VR Sink  InstantiateOnLoad=on  SampleTime=-1  ViewEnable=on  RemoteChange=off  RemoteView=off  FieldsWritten=Helicopter.rotation.4.1.1.double#Helicopter.translation.3.1.1.double  WorldFileName=quadrotor_world_ucart.wrl  AutoView=on  VideoDimensions=[]  AllowVariableSize=off
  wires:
  Bus Creator2/1 -> Bus Selector/1
  Demux/1 -> Bus Creator1/3
  Gain/1 -> Bus Creator1/2
  Gain2/1 -> Bus Creator1/1
  Rate Transition1/1 -> VR Sink/2
  Rate Transition/1 -> VR Sink/1
  Demux/3 -> Gain/1
  Demux/2 -> Gain2/1
  Bus Creator1/1 -> Gain1/1
  Bus Selector/1 -> Bus Creator/3  "<phi>"
  Bus Selector/3 -> Bus Creator/2  "<psi>"
  Bus Selector/2 -> Bus Creator/1  "<theta>"
  Gain1/1 -> Rate Transition1/1
  Demux1/3 -> Bus Creator2/3  "psi"
  Demux1/2 -> Bus Creator2/2  "theta"
  Demux1/1 -> Bus Creator2/1  "phi"
  Bus Creator/1 -> MATLAB Function/1(u)
  MATLAB Function/1(y) -> Rate Transition/1
  Displacement/1 -> Demux/1
  "Euler Angles "/1 -> Demux1/1

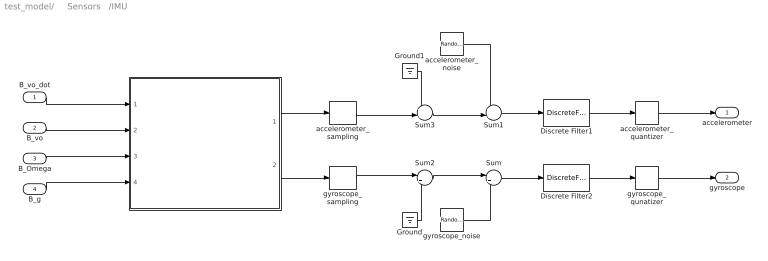
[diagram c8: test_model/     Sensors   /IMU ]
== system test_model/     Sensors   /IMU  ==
  B_vo_dot : Inport
  B_vo : Inport  Port=2
  B_Omega : Inport  Port=3
  B_g : Inport  Port=4
  " " : MATLAB Function  TreatAsAtomicUnit=on
  Discrete Filter1 : DiscreteFilter  Numerator=[0 0.749]  Denominator=[1 -0.251]  InitialStates=[0, 0, -1]  SampleTime=Tq
  Discrete Filter2 : DiscreteFilter  Numerator=[0 0.7327]  Denominator=[1 -0.2673]  SampleTime=Tq
  Ground : Ground
  Ground1 : Ground
  Sum : Sum  Inputs=|++
  Sum1 : Sum  Inputs=++|
  Sum2 : Sum  Inputs=|++
  Sum3 : Sum  Inputs=++|
  accelerometer_noise : RandomNumber  Mean=zeros(3,1)  Variance=[ 3e-7 ; 3.3e-7 ; 7.2e-7 ]  Seed=[0,1,2]  SampleTime=Tq
  accelerometer_quantizer : Quantizer  QuantizationInterval=2.4400e-04
  accelerometer_sampling : ZeroOrderHold  SampleTime=Tq
  gyroscope_noise : RandomNumber  Mean=zeros(3,1)  Variance=[ 2.2e-8 ; 1.1e-7 ; 2.4e-8 ]  Seed=[0,1,2]  SampleTime=Tq
  gyroscope_qunatizer : Quantizer  QuantizationInterval=1.1e-3
  gyroscope_sampling : ZeroOrderHold  SampleTime=Tq
  accelerometer : Outport
  gyroscope : Outport  Port=2
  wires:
  accelerometer_noise/1 -> Sum1/1
  Sum2/1 -> Sum/1
  Sum3/1 -> Sum1/2
  gyroscope_noise/1 -> Sum/2
  gyroscope_sampling/1 -> Sum2/1
  accelerometer_sampling/1 -> Sum3/2
  Ground/1 -> Sum2/2
  Ground1/1 -> Sum3/1
  B_vo_dot/1 -> " "/1(B_vo_dot)
  B_vo/1 -> " "/2(B_vo)
  B_Omega/1 -> " "/3(B_Omega)
  B_g/1 -> " "/4(B_g)
  " "/2(gyroReading) -> gyroscope_sampling/1
  " "/1(accelReading) -> accelerometer_sampling/1
  Sum1/1 -> Discrete Filter1/1
  Sum/1 -> Discrete Filter2/1
  accelerometer_quantizer/1 -> accelerometer/1
  gyroscope_qunatizer/1 -> gyroscope/1
  Discrete Filter1/1 -> accelerometer_quantizer/1
  Discrete Filter2/1 -> gyroscope_qunatizer/1

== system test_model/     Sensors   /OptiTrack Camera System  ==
  E_ro : Inport
  yaw : Inport  Port=2
  E_ro_noise : RandomNumber  Mean=zeros(3,1)  Variance=[ 7.9664e-10 ; 1.1928e-10 ; 5.0636e-10 ]  Seed=[0,1,2]  SampleTime=Tc
  E_ro_quantizer : Quantizer  QuantizationInterval=2.4400e-04
  E_ro_sampling : ZeroOrderHold  SampleTime=Tc
  Ground1 : Ground
  Ground2 : Ground
  Sum1 : Sum  Inputs=++|
  Sum3 : Sum  Inputs=++|
  Sum4 : Sum  Inputs=|++
  Sum6 : Sum  Inputs=|++
  yaw_noise : RandomNumber  Variance=1.0783e-9  SampleTime=Tq
  yaw_quantizer : Quantizer  QuantizationInterval=1.1e-3
  yaw_sampling : ZeroOrderHold  SampleTime=Tq
  E_ro_camera : Outport
  yaw_camera : Outport  Port=2
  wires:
  E_ro_noise/1 -> Sum1/1
  Sum3/1 -> Sum1/2
  Sum1/1 -> E_ro_quantizer/1
  E_ro_sampling/1 -> Sum3/2
  Ground1/1 -> Sum3/1
  Sum4/1 -> yaw_quantizer/1
  Sum6/1 -> Sum4/1
  yaw_noise/1 -> Sum4/2
  yaw_sampling/1 -> Sum6/1
  Ground2/1 -> Sum6/2
  yaw/1 -> yaw_sampling/1
  E_ro/1 -> E_ro_sampling/1
  E_ro_quantizer/1 -> E_ro_camera/1
  yaw_quantizer/1 -> yaw_camera/1

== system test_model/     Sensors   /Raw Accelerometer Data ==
  note: 1) Add Subsystem or Model blocks as valid variant choices. 2) You cannot connect blocks at this level. At simulation, connectivity is automatically determined, based on the active variant and port name matching.
  raw_accel_model : Inport
  Feedback : Subsystem  VariantControl=logAnalysisToggle==0
  "Raw Accelerometer Data " : Subsystem  VariantControl=logAnalysisToggle==1
  raw_accel : Outport

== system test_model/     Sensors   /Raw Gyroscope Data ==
  note: 1) Add Subsystem or Model blocks as valid variant choices. 2) You cannot connect blocks at this level. At simulation, connectivity is automatically determined, based on the active variant and port name matching.
  raw_gyro_model : Inport
  Feedback : Subsystem  VariantControl=logAnalysisToggle==0
  "Raw Gyroscope Data " : Subsystem  VariantControl=logAnalysisToggle==1
  raw_gyro : Outport

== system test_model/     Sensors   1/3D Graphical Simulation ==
  Displacement : Inport
  Euler Angles : Inport  Port=2
  Bus Creator : BusCreator  Inputs=3
  Bus Creator1 : BusCreator  Inputs=3
  Bus Creator2 : BusCreator  Inputs=3
  Bus Selector : BusSelector  OutputSignals=phi,theta,psi
  Demux : Demux  Outputs=3
  Demux1 : Demux  Outputs=3
  Gain : Gain  Gain=-1
  Gain1 : Gain  Gain=eye(3)*1  Multiplication=Matrix(K*u)
  Gain2 : Gain  Gain=-1
  MATLAB Function : MATLAB Function  TreatAsAtomicUnit=on
  Rate Transition : RateTransition  OutPortSampleTime=0.06
  Rate Transition1 : RateTransition  OutPortSampleTime=0.06
  VR Sink : vrlib/VR Sink  InstantiateOnLoad=on  SampleTime=-1  ViewEnable=on  RemoteChange=off  RemoteView=off  FieldsWritten=Helicopter.rotation.4.1.1.double#Helicopter.translation.3.1.1.double  WorldFileName=quadrotor_world_ucart.wrl  AutoView=on  VideoDimensions=[]  AllowVariableSize=off
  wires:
  Displacement/1 -> Demux/1
  Bus Creator2/1 -> Bus Selector/1
  Demux/1 -> Bus Creator1/3
  Gain/1 -> Bus Creator1/2
  Gain2/1 -> Bus Creator1/1
  Rate Transition1/1 -> VR Sink/2
  Rate Transition/1 -> VR Sink/1
  Demux/3 -> Gain/1
  Demux/2 -> Gain2/1
  Bus Creator1/1 -> Gain1/1
  Bus Selector/1 -> Bus Creator/3  "<phi>"
  Bus Selector/3 -> Bus Creator/2  "<psi>"
  Bus Selector/2 -> Bus Creator/1  "<theta>"
  Gain1/1 -> Rate Transition1/1
  Demux1/3 -> Bus Creator2/3  "psi"
  Demux1/2 -> Bus Creator2/2  "theta"
  Demux1/1 -> Bus Creator2/1  "phi"
  Euler Angles/1 -> Demux1/1
  Bus Creator/1 -> MATLAB Function/1(u)
  MATLAB Function/1(y) -> Rate Transition/1

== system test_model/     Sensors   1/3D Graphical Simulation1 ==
  "Euler Angles " : Inport
  Displacement : Inport  Port=2
  Bus Creator : BusCreator  Inputs=3
  Bus Creator1 : BusCreator  Inputs=3
  Bus Creator2 : BusCreator  Inputs=3
  Bus Selector : BusSelector  OutputSignals=phi,theta,psi
  Demux : Demux  Outputs=3
  Demux1 : Demux  Outputs=3
  Gain : Gain  Gain=-1
  Gain1 : Gain  Gain=eye(3)*1  Multiplication=Matrix(K*u)
  Gain2 : Gain  Gain=-1
  MATLAB Function : MATLAB Function  TreatAsAtomicUnit=on
  Rate Transition : RateTransition  OutPortSampleTime=0.06
  Rate Transition1 : RateTransition  OutPortSampleTime=0.06
  VR Sink : vrlib/VR Sink  InstantiateOnLoad=on  SampleTime=-1  ViewEnable=on  RemoteChange=off  RemoteView=off  FieldsWritten=Helicopter.rotation.4.1.1.double#Helicopter.translation.3.1.1.double  WorldFileName=quadrotor_world_ucart.wrl  AutoView=on  VideoDimensions=[]  AllowVariableSize=off
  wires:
  Bus Creator2/1 -> Bus Selector/1
  Demux/1 -> Bus Creator1/3
  Gain/1 -> Bus Creator1/2
  Gain2/1 -> Bus Creator1/1
  Rate Transition1/1 -> VR Sink/2
  Rate Transition/1 -> VR Sink/1
  Demux/3 -> Gain/1
  Demux/2 -> Gain2/1
  Bus Creator1/1 -> Gain1/1
  Bus Selector/1 -> Bus Creator/3  "<phi>"
  Bus Selector/3 -> Bus Creator/2  "<psi>"
  Bus Selector/2 -> Bus Creator/1  "<theta>"
  Gain1/1 -> Rate Transition1/1
  Demux1/3 -> Bus Creator2/3  "psi"
  Demux1/2 -> Bus Creator2/2  "theta"
  Demux1/1 -> Bus Creator2/1  "phi"
  Bus Creator/1 -> MATLAB Function/1(u)
  MATLAB Function/1(y) -> Rate Transition/1
  Displacement/1 -> Demux/1
  "Euler Angles "/1 -> Demux1/1

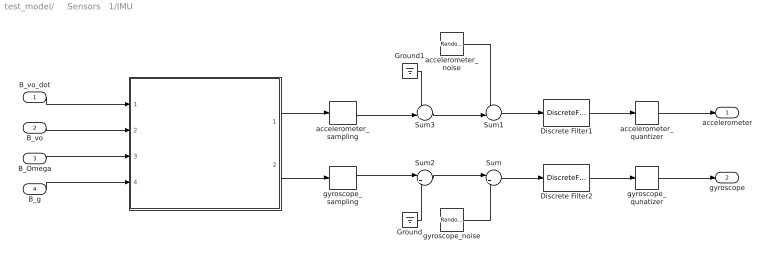
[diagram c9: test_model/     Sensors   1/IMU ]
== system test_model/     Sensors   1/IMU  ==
  B_vo_dot : Inport
  B_vo : Inport  Port=2
  B_Omega : Inport  Port=3
  B_g : Inport  Port=4
  " " : MATLAB Function  TreatAsAtomicUnit=on
  Discrete Filter1 : DiscreteFilter  Numerator=[0 0.749]  Denominator=[1 -0.251]  InitialStates=[0, 0, -1]  SampleTime=Tq
  Discrete Filter2 : DiscreteFilter  Numerator=[0 0.7327]  Denominator=[1 -0.2673]  SampleTime=Tq
  Ground : Ground
  Ground1 : Ground
  Sum : Sum  Inputs=|++
  Sum1 : Sum  Inputs=++|
  Sum2 : Sum  Inputs=|++
  Sum3 : Sum  Inputs=++|
  accelerometer_noise : RandomNumber  Mean=zeros(3,1)  Variance=[ 3e-7 ; 3.3e-7 ; 7.2e-7 ]  Seed=[0,1,2]  SampleTime=Tq
  accelerometer_quantizer : Quantizer  QuantizationInterval=2.4400e-04
  accelerometer_sampling : ZeroOrderHold  SampleTime=Tq
  gyroscope_noise : RandomNumber  Mean=zeros(3,1)  Variance=[ 2.2e-8 ; 1.1e-7 ; 2.4e-8 ]  Seed=[0,1,2]  SampleTime=Tq
  gyroscope_qunatizer : Quantizer  QuantizationInterval=1.1e-3
  gyroscope_sampling : ZeroOrderHold  SampleTime=Tq
  accelerometer : Outport
  gyroscope : Outport  Port=2
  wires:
  accelerometer_noise/1 -> Sum1/1
  Sum2/1 -> Sum/1
  Sum3/1 -> Sum1/2
  gyroscope_noise/1 -> Sum/2
  gyroscope_sampling/1 -> Sum2/1
  accelerometer_sampling/1 -> Sum3/2
  Ground/1 -> Sum2/2
  Ground1/1 -> Sum3/1
  B_vo_dot/1 -> " "/1(B_vo_dot)
  B_vo/1 -> " "/2(B_vo)
  B_Omega/1 -> " "/3(B_Omega)
  B_g/1 -> " "/4(B_g)
  " "/2(gyroReading) -> gyroscope_sampling/1
  " "/1(accelReading) -> accelerometer_sampling/1
  Sum1/1 -> Discrete Filter1/1
  Sum/1 -> Discrete Filter2/1
  accelerometer_quantizer/1 -> accelerometer/1
  gyroscope_qunatizer/1 -> gyroscope/1
  Discrete Filter1/1 -> accelerometer_quantizer/1
  Discrete Filter2/1 -> gyroscope_qunatizer/1

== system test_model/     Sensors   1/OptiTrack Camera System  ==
  E_ro : Inport
  yaw : Inport  Port=2
  E_ro_noise : RandomNumber  Mean=zeros(3,1)  Variance=[ 7.9664e-10 ; 1.1928e-10 ; 5.0636e-10 ]  Seed=[0,1,2]  SampleTime=Tc
  E_ro_quantizer : Quantizer  QuantizationInterval=2.4400e-04
  E_ro_sampling : ZeroOrderHold  SampleTime=Tc
  Ground1 : Ground
  Ground2 : Ground
  Sum1 : Sum  Inputs=++|
  Sum3 : Sum  Inputs=++|
  Sum4 : Sum  Inputs=|++
  Sum6 : Sum  Inputs=|++
  yaw_noise : RandomNumber  Variance=1.0783e-9  SampleTime=Tq
  yaw_quantizer : Quantizer  QuantizationInterval=1.1e-3
  yaw_sampling : ZeroOrderHold  SampleTime=Tq
  E_ro_camera : Outport
  yaw_camera : Outport  Port=2
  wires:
  E_ro_noise/1 -> Sum1/1
  Sum3/1 -> Sum1/2
  Sum1/1 -> E_ro_quantizer/1
  E_ro_sampling/1 -> Sum3/2
  Ground1/1 -> Sum3/1
  Sum4/1 -> yaw_quantizer/1
  Sum6/1 -> Sum4/1
  yaw_noise/1 -> Sum4/2
  yaw_sampling/1 -> Sum6/1
  Ground2/1 -> Sum6/2
  yaw/1 -> yaw_sampling/1
  E_ro/1 -> E_ro_sampling/1
  E_ro_quantizer/1 -> E_ro_camera/1
  yaw_quantizer/1 -> yaw_camera/1

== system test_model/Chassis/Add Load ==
  m_0 : Inport
  J_0 : Inport  Port=2
  r_oc_0 : Inport  Port=3
  m_l : Inport  Port=4
  J_l : Inport  Port=5
  r_ol : Inport  Port=6
  Add Load to Quadrotor : MATLAB Function  TreatAsAtomicUnit=on
  m : Outport
  J : Outport  Port=2
  r_oc : Outport  Port=3
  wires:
  r_ol/1 -> Add Load to Quadrotor/6(r_ol)
  Add Load to Quadrotor/3(r_oc) -> r_oc/1
  J_l/1 -> Add Load to Quadrotor/5(J_l)
  m_l/1 -> Add Load to Quadrotor/4(m_l)
  Add Load to Quadrotor/2(J) -> J/1
  r_oc_0/1 -> Add Load to Quadrotor/3(r_oc_0)
  J_0/1 -> Add Load to Quadrotor/2(J_0)
  Add Load to Quadrotor/1(m) -> m/1
  m_0/1 -> Add Load to Quadrotor/1(m_0)

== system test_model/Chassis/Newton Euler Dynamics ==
  F : Inport
  Q : Inport  Port=2
  v : Inport  Port=3
  Omega : Inport  Port=4
  m : Inport  Port=5
  J : Inport  Port=6
  r_oc : Inport  Port=7
  Newton-Euler Rigid Body Dynamics : MATLAB Function  TreatAsAtomicUnit=on
  dv : Outport
  dOmega : Outport  Port=2
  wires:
  m/1 -> Newton-Euler Rigid Body Dynamics/5(m)
  J/1 -> Newton-Euler Rigid Body Dynamics/6(J)
  r_oc/1 -> Newton-Euler Rigid Body Dynamics/7(r_oc)
  F/1 -> Newton-Euler Rigid Body Dynamics/1(F)
  Q/1 -> Newton-Euler Rigid Body Dynamics/2(Q)
  v/1 -> Newton-Euler Rigid Body Dynamics/3(v)
  Omega/1 -> Newton-Euler Rigid Body Dynamics/4(Omega)
  Newton-Euler Rigid Body Dynamics/1(dv) -> dv/1
  Newton-Euler Rigid Body Dynamics/2(dOmega) -> dOmega/1
